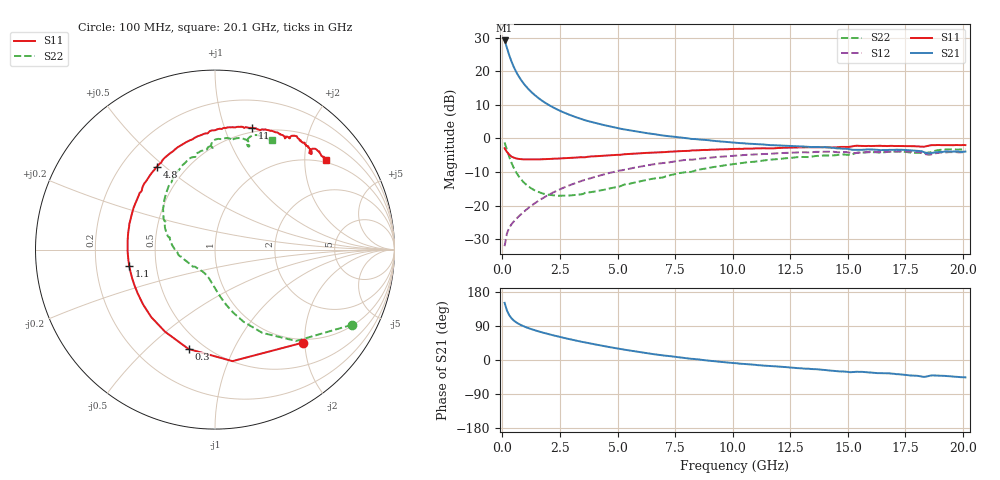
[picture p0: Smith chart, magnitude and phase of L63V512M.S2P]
!  Infineon Technologies AG
! BFR380L3 , PF131585-7, No.6, Th 09.10.01, soldered on pcb-board, measured with PP GSG850
!  Vce=3.5 V,  Ic=12.5 mA
! Common Emitter S-Parameters:  15. November 2001
#  GHz  S  MA  R  50
! f  S11  S21  S12  S22
! GHz  Mag  Ang  Mag  Ang  Mag  Ang  Mag  Ang
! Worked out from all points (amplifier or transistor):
!   201 points, 100 MHz to 20.1 GHz, reference 50 ohm
!   highest |S21| = 29.2 dB at 100 MHz (marker M1)
!   |S21| within 3 dB of that: start of sweep to 236.2 MHz
!   unconditionally stable (mu >= 1): 1.696 GHz to 4.453 GHz
!   at 3.4 GHz: K = 1.02, MAG = 8.4 dB, |S12| = -12.7 dB
!   at 10.1 GHz: K = 0.95, MSG = 1.9 dB, |S12| = -5.1 dB
!   at 20.1 GHz: K = 0.99, MSG = 0.1 dB, |S12| = -4.1 dB
!   S11 on the Smith chart (normalised r, x): 100 MHz: 0.93, -1.96; 300 MHz: 0.41, -0.68; 1.1 GHz: 0.35, -0.08; 4.8 GHz: 0.35, +0.47; 11 GHz: 0.46, +1.24; 20.1 GHz: 0.93, +2.52
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0.1  0.7137 -46.6  28.69 150.8  0.0249 68.7  0.8704 -28.8
0.2  0.629 -81.1  22.24 130.7  0.03841 57.5  0.681 -48.4
0.3  0.5731 -104.9  17.31 118.3  0.04681 52.6  0.5332 -60.4
0.4  0.5355 -121.4  13.92 110.1  0.05272 50.6  0.4326 -68.4
0.5  0.5173 -133.4  11.52 104.1  0.05809 51.1  0.3631 -74.1
0.6  0.504 -142.7  9.805 99.5  0.06328 51.7  0.314 -78.5
0.7  0.4955 -149.9  8.531 95.7  0.06852 52.9  0.2771 -82.2
0.8  0.4911 -155.9  7.532 92.5  0.07374 54.1  0.2492 -85.3
0.9  0.4885 -160.9  6.743 89.7  0.07907 55.0  0.2276 -88.0
1.1  0.4863 -169.1  5.584 84.9  0.09035 56.7  0.1974 -93.2
1.3  0.486 -175.7  4.761 80.7  0.1017 58.0  0.1767 -97.6
1.5  0.4869 178.5  4.159 76.8  0.1136 58.8  0.163 -101.9
2  0.4939 167.1  3.171 68.4  0.144 59.2  0.1452 -112.4
2.6  0.5048 156.1  2.489 59.4  0.1809 58.1  0.1403 -124.7
3.5  0.5232 141.7  1.908 47.4  0.2369 54.4  0.1488 -140.5
4.8  0.5643 125.0  1.476 32.4  0.3143 47.4  0.1839 -164.5
6.8  0.6224 103.8  1.128 13.5  0.4236 34.5  0.2595 166.1
10.1  0.6975 78.6  0.8622 -8.2  0.5536 13.0  0.4175 130.6
11  0.7074 73.1  0.8244 -12.8  0.5798 7.2  0.4527 122.0
13.5  0.7365 60.7  0.7449 -24.1  0.6255 -8.1  0.5403 101.2
16.8  0.7728 48.4  0.6755 -35.2  0.6332 -24.5  0.6319 79.1
20.1  0.7948 39.0  0.6369 -45.8  0.6262 -38.4  0.6884 62.3
